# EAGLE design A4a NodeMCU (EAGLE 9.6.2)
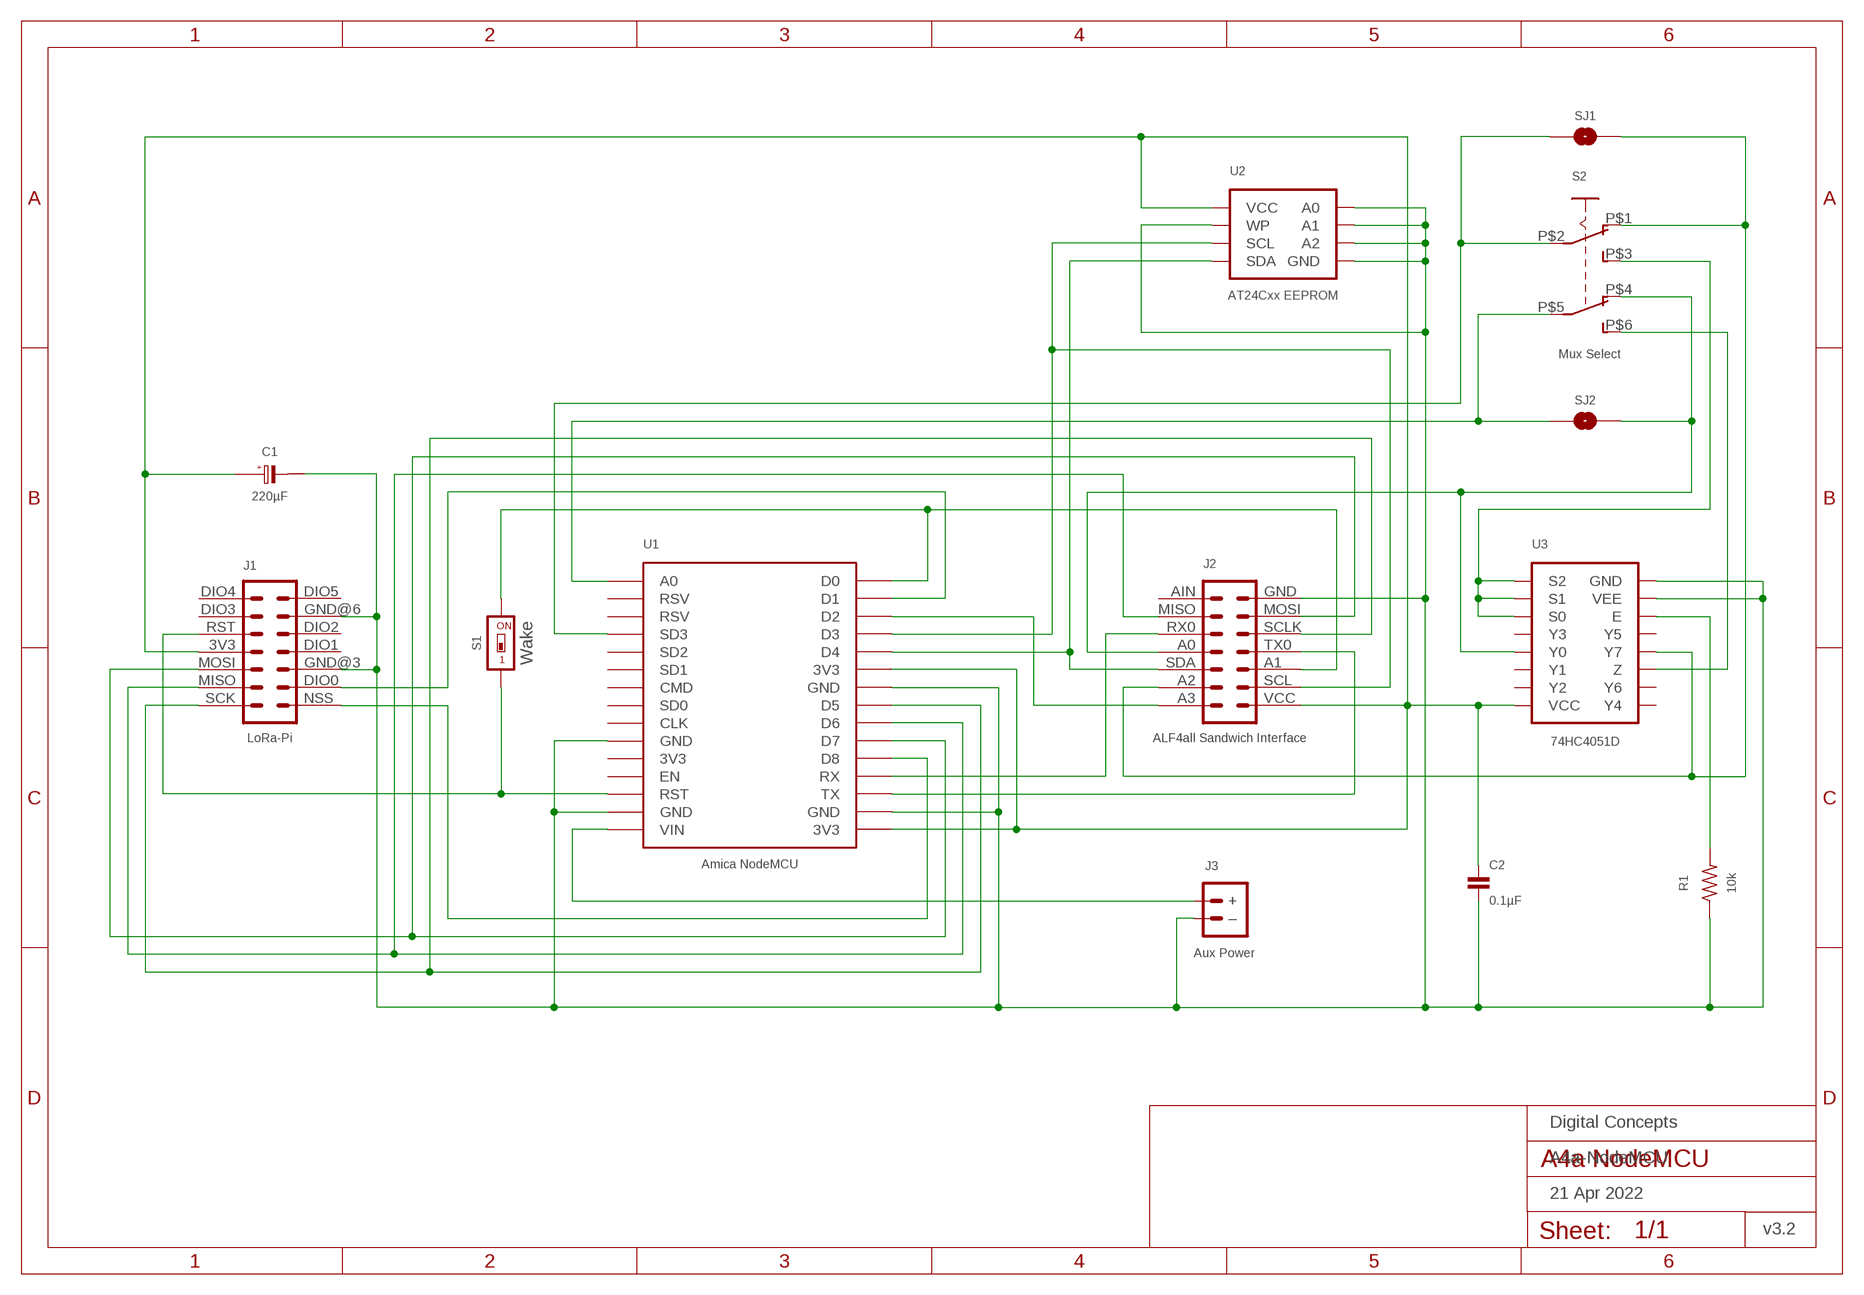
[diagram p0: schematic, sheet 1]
FRAME1 (A4L-LOC): DATE: 21 Apr 2022; OWNER: Digital Concepts; TITLE: A4a-NodeMCU; VERSION: v3.2

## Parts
C1  220µF  CAPACITOR-TANTALUM-3528  [C3528-21]
C2  0.1µF  CAPACITOR-0805  [C0805]
J1  LoRa-Pi  RFM95W-PI-HEADER  [RFM95W-PI]
J2  ALF4all Sandwich Interface  HEADER-2X7-ALF4ALL-PROCESSOR-B  [CONN_2X7-ALF4ALL-PROCESSOR-B]
J3  Aux Power  JST-PH2.0-2-MALE-HORIZONTALJST-PTH-2  [JST-PH2.0-2-HORIZONTAL]
R1  10k  RESISTORR0805  [R0805]
S1  Wake  SWITCH-DIP-SWS001  [SMD-001]
S2  Mux Select  SWITCH-DPDT  [SWITCH-DPDT-SMD]
SJ1  SJ  [SJ]
SJ2  SJ  [SJ]
U1  Amica NodeMCU  AMICA-NODEMCU  [AMICA-NODEMCU]
U2  AT24Cxx EEPROM  AT24CXX-EEPROM  [SOP-8]
U3  74HC4051D  [SOP16]

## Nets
GND: C1.2(-) C2.2 J1.GND@3 J1.GND@6 J2.GND J3.-(–) R1.1 U1.GND@2(GND) U1.GND@9(GND) U1.GND@25(GND) U1.GND@29(GND) U2.P$1(A0) U2.P$2(A1) U2.P$3(A2) U2.P$4(GND) U2.P$7(WP) U3.7(VEE) U3.8(GND)
N$1: S2.P$5(P2) SJ2.1 U1.A0
N$2: J2.A3 U1.D2
N$3: J2.A1 S1.2 U1.D0
N$4: J1.RST S1.1 U1.RST
N$5: J2.A0 S2.P$4(O2) SJ2.2 U3.13(Y0)
N$6: J1.SCK J2.SCLK U1.D5
N$7: J2.RX0 U1.RX
N$8: R1.2 U3.6(E)
N$9: J3.+ U1.VIN
N$10: J2.SDA U1.D4 U2.P$5(SDA)
N$11: J2.SCL U1.D3 U2.P$6(SCL)
N$12: J1.MISO J2.MISO U1.D6
N$13: J1.MOSI J2.MOSI U1.D7
N$14: J2.TX0 U1.TX
N$15: J1.NSS U1.D8
N$16: S2.P$3(S1) U3.9(S2) U3.10(S1) U3.11(S0)
N$17: J1.DIO0 U1.D1
N$18: S2.P$2(P1) SJ1.1 U1.SD3
N$19: S2.P$6(S2) U3.3(Z)
N$20: J2.A2 S2.P$1(O1) SJ1.2 U3.4(Y7)
VCC: C1.1(+) C2.1 J1.3V3 J2.VCC U1.3V3@1(3V3) U1.3V3@10(3V3) U2.P$8(VCC) U3.16(VCC)
Unconnected: J1.DIO1 J1.DIO2 J1.DIO3 J1.DIO4 J1.DIO5 J2.AIN U1.3V3@26(3V3) U1.CLK U1.CMD U1.EN U1.RSV@17(RSV) U1.RSV@18(RSV) U1.SD0 U1.SD1 U1.SD2 U3.1(Y4) U3.2(Y6) U3.5(Y5) U3.12(Y3) U3.14(Y1) U3.15(Y2)

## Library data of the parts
C1 = digitalconcepts:CAPACITOR-TANTALUM-3528: Capacitor Polarised EIA 3528-21 (KEMET B)
C2 = digitalconcepts:CAPACITOR-0805: 0805 Capacitor
J1 = digitalconcepts:RFM95W-PI-HEADER: RFM95W LoRa Wireless Transceiver Raspberry Pi Daughter Board
J2 = digitalconcepts:HEADER-2X7-ALF4ALL-PROCESSOR-B: ALF4all 'Sandwich' Processor (Bottom) 2x7 Pin Header Header soldered to underside of PCB
J3 = digitalconcepts:JST-PH2.0-2-MALE-HORIZONTAL: Multi connection point. Often used as Generic Header-pin footprint for 0.1 inch spaced/style header connections; PROD_ID: CONN-09863; SKU: PRT-09914
R1 = digitalconcepts:RESISTOR: Resistor; SPICEPREFIX: R
S1 = digitalconcepts:SWITCH-DIP-SWS001: SMD Dip Switch 1 pol.
S2 = digitalconcepts:SWITCH-DPDT: Switch SMD DPDT
SJ1 SJ2 = digitalconcepts:SJ: Solder Jumper
U1 = digitalconcepts:AMICA-NODEMCU: Amica NodeMCU Development Board
U2 = digitalconcepts:AT24CXX-EEPROM: AT24Cxx EEPROM SOP-8
U3 = digitalconcepts:74HC4051D: 74HC4051 8-Port Multiplexer SOP-16

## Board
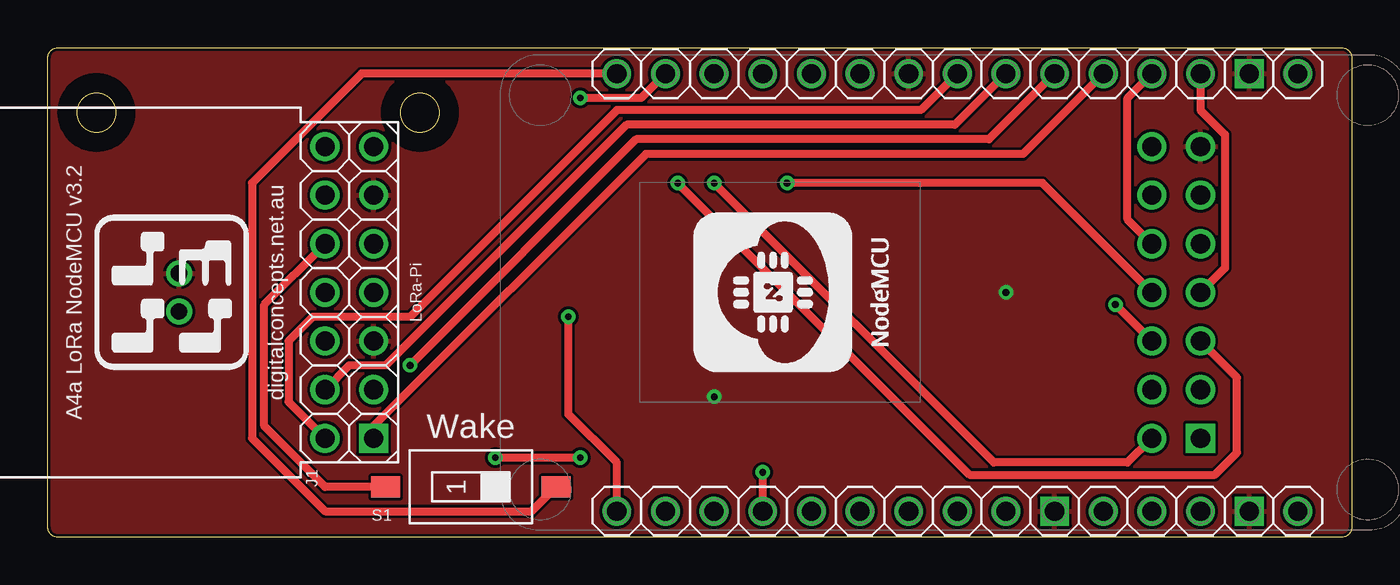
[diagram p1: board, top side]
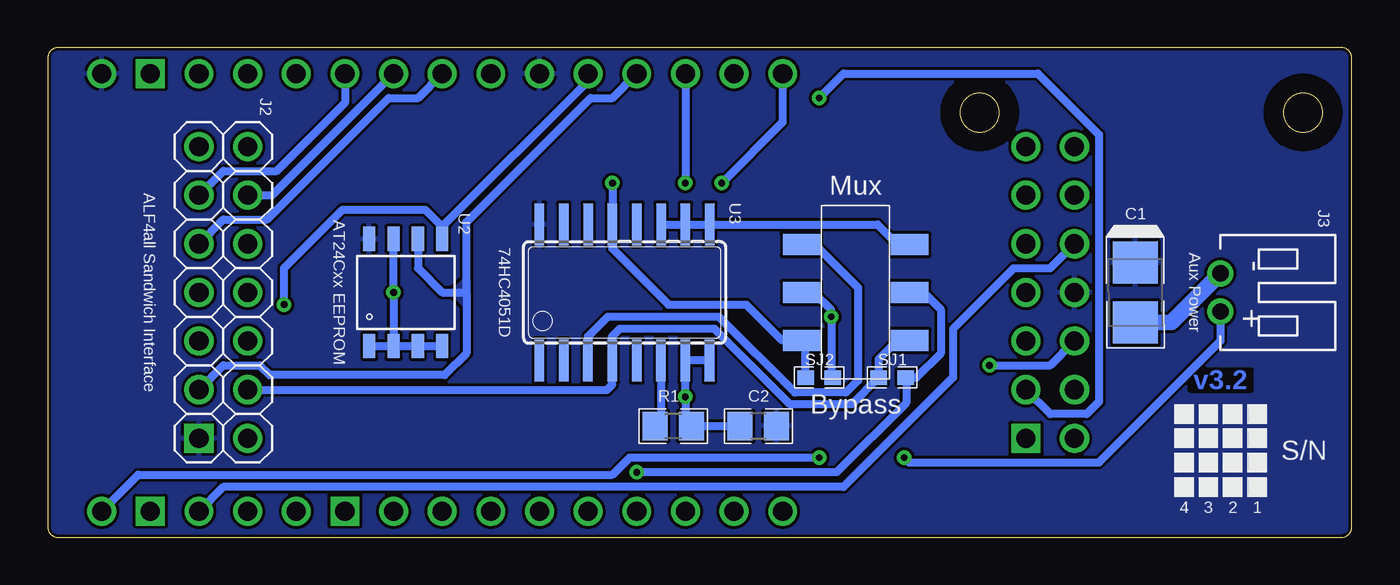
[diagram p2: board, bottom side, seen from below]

Size 68.08 x 25.56 mm. Coordinates in mm from the lower left corner, seen from the top.
Outline: 87 segments
Outline: circle at 19.42,22.18 radius 1.02
Outline: circle at 2.53,22.18 radius 1.02
Copper layers (1*16): Top 0.035mm / dielectric 1.5mm / Bottom 0.035mm
Design rules "default *": minimum track width 6mil, minimum drill 0.35mm, track to track 6mil, track to pad 6mil, pad to pad 6mil, via to via 6mil, smd to smd 6mil, copper to edge 6mil, drill to drill 6mil, minimum pad ring 10mil, minimum via ring 8mil, stop-mask expansion 4mil, vias tented up to drill 0mil, thermal gap 6mil

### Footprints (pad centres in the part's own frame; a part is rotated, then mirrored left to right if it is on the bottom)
C3528-21 = smd 2.21 x 2.35: 1 -1.565,0; 2 1.565,0
C0805 = smd 1.3 x 1.5: 1 -0.95,0; 2 0.95,0
RFM95W-PI = drill 1 pad 1.524: 3V3 7.62,2.54; DIO0 2.54,0; DIO1 7.62,0; DIO2 10.16,0; DIO3 12.7,2.54; DIO4 15.24,2.54; DIO5 15.24,0; GND@3 5.08,0; GND@6 12.7,0; MISO 2.54,2.54; MOSI 5.08,2.54; RST 10.16,2.54; SCK 0,2.54 | drill 1 pad 1.524 square: NSS 0,0
CONN_2X7-ALF4ALL-PROCESSOR-B = drill 1 pad 1.524: A0 7.62,2.54; A1 5.08,0; A2 2.54,2.54; A3 0,2.54; AIN 15.24,2.54; GND 15.24,0; MISO 12.7,2.54; MOSI 12.7,0; RX0 10.16,2.54; SCL 2.54,0; SCLK 10.16,0; SDA 5.08,2.54; TX0 7.62,0 | drill 1 pad 1.524 square: VCC 0,0
JST-PH2.0-2-HORIZONTAL = drill 0.85: + 1,0; - -1,0
R0805 = smd 1.3 x 1.5: 1 -0.95,0; 2 0.95,0
SMD-001 = smd 1.1 x 1.5: 1 0,-4.45; 2 0,4.45
SWITCH-DPDT-SMD = smd 1.95 x 1.1: P$1 -2.825,2.5; P$2 -2.825,0; P$3 -2.825,-2.5; P$4 2.825,2.5; P$5 2.825,0; P$6 2.825,-2.5
SJ = smd 0.864 x 0.762: 1 -0.711,0; 2 0.711,0
AMICA-NODEMCU = drill 1: 3V3@1 0,0; 3V3@10 0,22.86; 3V3@26 -22.86,10.16; A0 -22.86,35.56; CLK -22.86,15.24; CMD -22.86,20.32; D0 0,35.56; D1 0,33.02; D2 0,30.48; D3 0,27.94; D4 0,25.4; D5 0,17.78; D6 0,15.24; D7 0,12.7; D8 0,10.16; EN -22.86,7.62; GND@9 0,20.32; RST -22.86,5.08; RSV@17 -22.86,33.02; RSV@18 -22.86,30.48; RX 0,7.62; SD0 -22.86,17.78; SD1 -22.86,22.86; SD2 -22.86,25.4; SD3 -22.86,27.94; TX 0,5.08; VIN -22.86,0 | drill 1 square: GND@2 0,2.54; GND@25 -22.86,12.7; GND@29 -22.86,2.54
SOP-8 = smd 0.635 x 1.27: P$1 -1.905,-2.794; P$2 -0.635,-2.794; P$3 0.635,-2.794; P$4 1.905,-2.794; P$5 1.905,2.794; P$6 0.635,2.794; P$7 -0.635,2.794; P$8 -1.905,2.794
SOP16 = smd 0.5 x 2.2: 1 -4.445,-3.55; 2 -3.185,-3.55; 3 -1.915,-3.55; 4 -0.645,-3.55; 5 0.635,-3.55; 6 1.895,-3.55; 7 3.165,-3.55; 8 4.435,-3.55; 9 4.445,3.55; 10 3.175,3.55; 11 1.905,3.55; 12 0.635,3.55; 13 -0.635,3.55; 14 -1.905,3.55; 15 -3.175,3.55; 16 -4.445,3.55

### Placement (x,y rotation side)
C1  11.29,12.78 270.1 bottom
C2  30.98,5.8 180 bottom
J1  17.01,5.16 90 top
J2  60.19,5.16 90 top
J3  6.85,12.78 270 bottom
R1  35.42,5.8 180 bottom
S1  22.09,2.62 270 top
S2  25.9,12.78 180 bottom
SJ1  23.99,8.34 180 bottom
SJ2  27.8,8.34 180 bottom
U1  65.27,24.21 90 top
U2  49.39,12.78 0 bottom
U3  37.96,12.78 0 bottom

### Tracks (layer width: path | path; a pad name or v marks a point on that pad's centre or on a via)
$X1
  cutout Top: 2.53,24.21 arc180 2.53,20.15 arc180
$X2
  cutout Bottom: 2.53,24.21 arc180 2.53,20.15 arc180
$X3
  cutout Top: 19.42,24.21 arc180 19.42,20.15 arc180
$X4
  cutout Bottom: 19.42,24.21 arc180 19.42,20.15 arc180
GND  (via drill 0.35)
  Bottom 0.406: U2.P$1 U2.P$2 | U2.P$7 v50.03,12.78 U2.P$2 | U3.8 U3.7 34.8,7.34 v34.79,7.33 34.79,6.11 R1.1 C2.2 | U2.P$2 U2.P$3 U2.P$4
  Bottom 0.813: C1.2 9.41,11.22 J3.-
  pour Top (rank 5): -2.04,27.39 70.35,27.39 70.35,-1.82 -2.04,-1.82
N$1  (via drill 0.35)
  Top 0.406: U1.A0 29.71,3.89 27.17,6.43 v27.17,11.51
  Bottom 0.406: S2.P$5 28.09,12.78 27.17,11.86 v27.17,11.51 27.17,8.41 SJ2.1
N$2  (via drill 0.35)
  Top 0.406: v34.79,18.5 49.39,3.89 56.38,3.89 J2.A3
  Bottom 0.406: U1.D2 v34.79,18.5
N$3  (via drill 0.35)
  Top 0.406: U1.D0 16.37,24.21 10.66,18.5 10.66,5.16 14.47,1.35 25.27,1.35 S1.2 | v32.88,18.5 48.12,3.26 60.95,3.26 62.09,4.41 62.09,8.34 J2.A1
  Bottom 0.406: U1.D0 29.71,21.67 v32.88,18.5
N$4
  Top 0.406: S1.1 14.47,2.62 11.29,5.8 11.29,12.15 J1.RST
  Bottom 0.406: U1.RST 58.92,2.62 26.53,2.62 20.82,8.34 20.82,10.88 17.64,14.05 15.74,14.05 J1.RST
N$5  (via drill 0.35)
  Top 0.406: J2.A0 51.93,18.5 v38.6,18.5
  Bottom 0.406: v38.6,18.5 U3.13 38.6,15.07 35.68,12.15 31.61,12.15 29.75,10.28 S2.P$4 28.51,10.07 SJ2.2
N$6
  Top 0.406: U1.D5 45.58,22.31 29.71,22.31 18.91,11.51 13.83,11.51 12.56,10.24 12.56,7.07 J1.SCK
  Bottom 0.406: J2.SCLK 58.92,16.59 56.63,16.59 50.28,22.94 48.76,22.94 U1.D5
N$7
  Top 0.406: U1.RX 56.38,22.94 56.38,16.59 J2.RX0
N$8
  Bottom 0.406: U3.6 36.07,6.1 R1.2
N$9  (via drill 0.35)
  Top 0.406: v27.8,4.15 v23.36,4.15
  Bottom 0.406: U1.VIN 63.36,3.26 38.6,3.26 37.71,4.15 v27.8,4.15 | J3.+ 6.85,10.24 13.2,3.89 23.1,3.89 v23.36,4.15
N$10  (via drill 0.35)
  Top 0.406: J2.SDA v55.74,12.15
  Bottom 0.406: U1.D4 39.87,23.83 47.49,16.21 | U2.P$5 47.49,16.21 | 47.49,16.21 48.38,17.1 52.7,17.1 55.74,14.05 v55.74,12.15
N$11
  Bottom 0.406: J2.SCL 58.92,8.97 57.01,8.97 56.51,8.46 47.36,8.46 46.22,9.61 46.22,12.78 | U2.P$6 48.76,14.05 47.49,12.78 46.22,12.78 | U1.D3 38.6,22.94 39.74,22.94 46.22,16.47 46.22,12.78
  pour Bottom: 46.85,12.78 46.22,13.42 46.22,12.15
N$12
  Top 0.406: U1.D6 47.36,21.55 30.22,21.55 17.64,8.97 15.74,8.97 J1.MISO
  Bottom 0.406: J2.MISO 56.38,17.86 U1.D6
N$13  (via drill 0.35)
  Top 0.406: U1.D7 49.14,20.78 30.72,20.78 v18.91,8.97
  Bottom 0.406: J2.MOSI 58.92,19.13 56.12,19.13 52.57,22.69 U1.D7 | v18.91,8.97 15.74,8.97 J1.MOSI
N$14
  Top 0.406: U1.TX 60.19,22.31 61.46,21.04 61.46,14.05 J2.TX0
N$15
  Top 0.406: U1.D8 50.92,20.02 31.23,20.02 17.01,5.8 J1.NSS
N$16
  Bottom 0.406: U3.11 U3.10 U3.9 24.76,16.33 23.71,15.28 S2.P$3
N$17  (via drill 0.35)
  Top 0.406: U1.D1 30.98,22.94 v27.8,22.94
  Bottom 0.406: J1.DIO0 15.74,6.43 13.83,6.43 13.2,7.07 13.2,21.04 16.37,24.21 26.53,24.21 v27.8,22.94
N$18  (via drill 0.35)
  Top 0.406: U1.SD3 v37.33,3.38
  Bottom 0.406: S2.P$2 22.34,12.78 21.45,11.89 21.45,9.61 22.72,8.34 SJ1.1 23.26,8.31 23.26,7.02 26.89,3.38 v37.33,3.38
N$19
  Bottom 0.406: U3.3 39.88,10.49 38.85,11.51 33.04,11.51 29.07,7.55 26.41,7.55 25.77,8.19 25.77,13.04 28.02,15.28 S2.P$6
N$20
  Bottom 0.406: J2.A2 38.87,7.7 38.61,7.96 U3.4 38.61,10.49 38.22,10.88 33.26,10.88 29.33,6.94 26.1,6.94 SJ1.2 24.7,9.29 23.71,10.28 S2.P$1
VCC
  pour Bottom (rank 5): -0.77,26.12 69.08,26.12 69.08,-0.55 -0.77,-0.55

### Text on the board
Bottom: v3.2
tPlace: A4a LoRa NodeMCU v3.2 | digitalconcepts.net.au
bPlace: S/N | 1 | 2 | 3 | 4
bNames: Mux | Bypass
